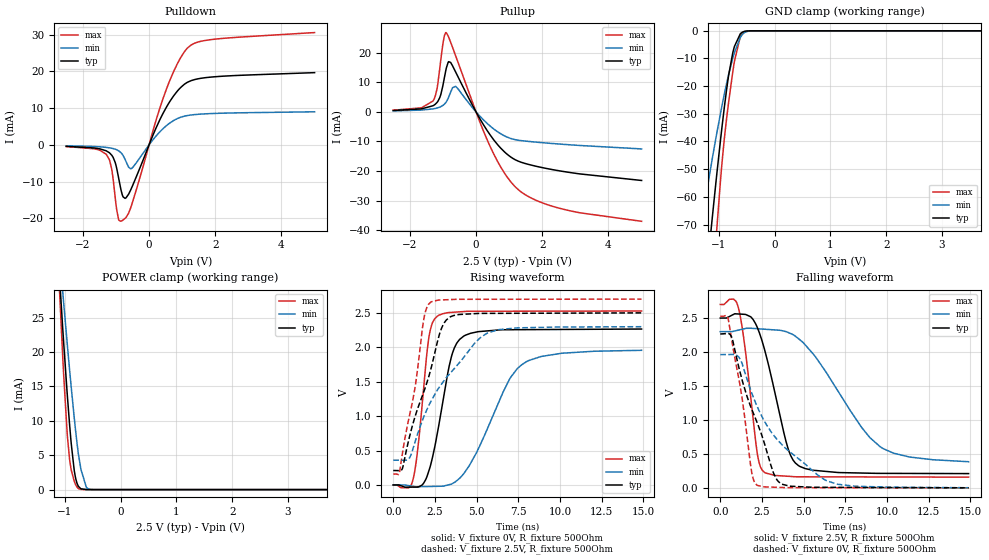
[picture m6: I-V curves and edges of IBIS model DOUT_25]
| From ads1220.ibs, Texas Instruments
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|   DOUT_25 Model
[Model]   DOUT_25
Model_type   3-state
Polarity   Non-Inverting
Vmeas = 1.25
Vref = 1.25
Cref = 15pF
Rref = 500
|   typ   min   max
|   (nom PVT)   (Fast PVT)   (slow PVT)
C_comp   3.058p   2.545p   3.580p
|C_comp (ON state)   3.149p   2.639p   3.673p
|C_comp (OFF state)   3.058p   2.545p   3.580p
| Where   nom PVT is  Nominal Process, 2.5V, 27C
|   Fast PVT is Strong Process, 2.7V, -40C
|   Slow PVT is Weak Process, 2.3V, 125C
[Voltage Range]   2.5   2.3   2.7
[Temperature Range]   27   125   -40
[Pullup Reference]   2.5   2.3   2.7
[Pulldown Reference]   0   0   0
[Power Clamp Reference]   2.5   2.3   2.7
[GND Clamp Reference]   0   0   0
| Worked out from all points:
|   slope of the pulldown table from 0 to 0.375 V, typ, clamps not added: 48.4 ohm
|   slope of the pullup table from 0 to 0.375 V, typ, clamps not added: 54 ohm
|   GND clamp passes 1 mA (typ) near -0.61 V on its own axis
|   POWER clamp passes 1 mA (typ) near -0.79 V on its own axis
|   falling waveform, V_fixture 2.5V, R_fixture 500Ohm: 20-80 % time 1.31ns typ, 3.14ns min, 720ps max; typ from 2.5 V to 0.21 V
|   rising waveform, V_fixture 0V, R_fixture 500Ohm: 20-80 % time 1.04ns typ, 2.23ns min, 608ps max; typ from 0 V to 2.27 V
|   rising waveform, V_fixture 2.5V, R_fixture 500Ohm: 20-80 % time 1.67ns typ, 2.95ns min, 1.02ns max; typ from 0.21 V to 2.5 V
|   falling waveform, V_fixture 0V, R_fixture 500Ohm: 20-80 % time 1.81ns typ, 3.22ns min, 936ps max; typ from 2.27 V to 0 V
[Pulldown]
|   Voltage   I(typ)   I(min)   I(max)
-2.5V     -374.4uA   -222uA     -428.3uA
-1.285V   -1.63mA    -664.6uA   -2.642mA
-1.127V   -2.768mA   -891.6uA   -6.533mA
-1.022V   -4.749mA   -1.148mA   -14.24mA
-917.5mV  -8.99mA    -1.591mA   -20.32mA
-850mV    -12.08mA   -2.077mA   -20.77mA
-722.5mV  -14.53mA   -3.925mA   -19.97mA
-535mV    -11.86mA   -6.426mA   -16.59mA
432.5mV   8.759mA    4.52mA     12.87mA
1.167V    17.09mA    8.023mA    26.44mA
1.903V    18.5mA     8.556mA    28.7mA
5V        19.68mA    9.028mA    30.59mA
[GND Clamp]
|   Voltage   I(typ)   I(min)   I(max)
-2.5V     -381.2mA   -244.6mA   -533.1mA
-1.33V    -111.2mA   -71.95mA   -159mA
-1.225V   -88.94mA   -58.76mA   -126.6mA
-1.135V   -70.54mA   -47.94mA   -99.39mA
-1.038V   -51.48mA   -36.82mA   -71.24mA
-910mV    -28.65mA   -23.46mA   -40.16mA
-827.5mV  -16.19mA   -15.83mA   -25.91mA
-722.5mV  -5.622mA   -7.819mA   -10.98mA
-617.5mV  -1.084mA   -2.441mA   -2.106mA
-572.5mV  -410.6uA   -1.162mA   -730.1uA
-325mV    -375.7nA   -5.011uA   -154.3nA
5V        0A         0A         0A
[Pullup]
|   Voltage   I(typ)   I(min)   I(max)
-2.5V     452.7uA    310.9uA    552.2uA
-1.3V     2.066mA    1.006mA    3.662mA
-1.18V    3.146mA    1.29mA     7.679mA
-1.09V    4.964mA    1.628mA    15.15mA
-992.5mV  9.333mA    2.245mA    23.56mA
-895mV    14.87mA    3.435mA    26.72mA
-767.5mV  16.7mA     6.64mA     23.55mA
-617.5mV  13.5mA     8.634mA    19mA
432.5mV   -7.889mA   -4.855mA   -11.84mA
1.19V     -16.21mA   -9.414mA   -25.38mA
2.428V    -19.75mA   -10.8mA    -32.28mA
5V        -23.18mA   -12.52mA   -36.97mA
[POWER Clamp]
|   Voltage   I(typ)   I(min)   I(max)
-2.5V     236.5mA    191.7mA    294.3mA
-1.143V   36.82mA    38.8mA     36.45mA
-1.045V   24.03mA    29.22mA    20.05mA
-1.03V    22.16mA    27.79mA    17.7mA
-962.5mV  14.22mA    21.5mA     8.459mA
-917.5mV  9.478mA    17.47mA    4.401mA
-835mV    2.87mA     10.54mA    1.255mA
-760mV    481uA      5.211mA    158.7uA
-715mV    118.5uA    2.983mA    26.06uA
-617.5mV  4.222uA    344.5uA    596.9nA
-535mV    257.6nA    35.27uA    3.063nA
5V        0A         0A         0A
[Ramp]
R_load = 500
|   typ   min   max
dV/dt_r   1.35931/1.03236e-09   1.17388/2.22345e-09   1.51637/6.05571e-10
dV/dt_f   1.37395/1.3112e-09   1.14911/3.12849e-09   1.52529/7.18066e-10
[Falling Waveform]
V_fixture = 2.5V
V_fixture_min = 2.3V
V_fixture_max = 2.7V
R_fixture = 500Ohm
C_fixture = 0F
|   Time   V(typ)   V(min)   V(max)
0s        2.5V       2.3V       2.7V
793ps     2.554V     2.306V     2.779V
1.097ns   2.56V      2.323V     2.644V
1.506ns   2.554V     2.347V     2.023V
2.23ns    2.358V     2.343V     494.4mV
2.65ns    2.044V     2.336V     228.9mV
4.054ns   591.3mV    2.29V      170.7mV
4.741ns   320.5mV    2.187V     162.9mV
9.584ns   213.4mV    607.9mV    160.5mV
14.9ns    210.1mV    384.8mV    157.8mV
[Rising Waveform]
V_fixture = 0V
V_fixture_min = 0V
V_fixture_max = 0V
R_fixture = 500Ohm
C_fixture = 0F
|   Time   V(typ)   V(min)   V(max)
0s        2.773nV    5.389nV    2.124nV
1.183ns   -31.49mV   -19.91mV   75.87mV
1.534ns   -26.2mV    -25.63mV   657.9mV
2.121ns   193.6mV    -22.45mV   2.115V
2.65ns    756.5mV    -19.58mV   2.453V
3.524ns   1.892V     16.37mV    2.508V
4.311ns   2.173V     192.8mV    2.521V
6.971ns   2.256V     1.534V     2.524V
7.704ns   2.256V     1.746V     2.525V
14.9ns    2.266V     1.956V     2.527V
[Rising Waveform]
V_fixture = 2.5V
V_fixture_min = 2.3V
V_fixture_max = 2.7V
R_fixture = 500Ohm
C_fixture = 0F
|   Time   V(typ)   V(min)   V(max)
0s        209.9mV    359.5mV    157.8mV
373.6ps   208.2mV    359.4mV    176.6mV
557.4ps   243.1mV    359.3mV    469.5mV
991.5ps   715mV      398.6mV    1.026V
1.361ns   1.033V     665.4mV    1.502V
1.849ns   1.364V     998.3mV    2.428V
2.249ns   1.678V     1.208V     2.656V
3.178ns   2.395V     1.557V     2.691V
5.719ns   2.493V     2.214V     2.698V
14.9ns    2.5V       2.299V     2.7V
[Falling Waveform]
|Gnd
V_fixture = 0V
V_fixture_min = 0V
V_fixture_max = 0V
R_fixture = 500Ohm
C_fixture = 0F
|   Time   V(typ)   V(min)   V(max)
0s        2.266V     1.962V     2.527V
482.9ps   2.272V     1.963V     2.483V
704.4ps   2.209V     1.964V     2.153V
1.213ns   1.681V     1.888V     1.469V
1.882ns   1.162V     1.403V     237.9mV
2.194ns   971.9mV    1.21V      41.64mV
3.212ns   208.5mV    772.9mV    9.542mV
3.694ns   54.44mV    638.9mV    5.525mV
7.045ns   7.277mV    52.87mV    2.194mV
14.9ns    57.73uV    2.12mV     50.27nV
